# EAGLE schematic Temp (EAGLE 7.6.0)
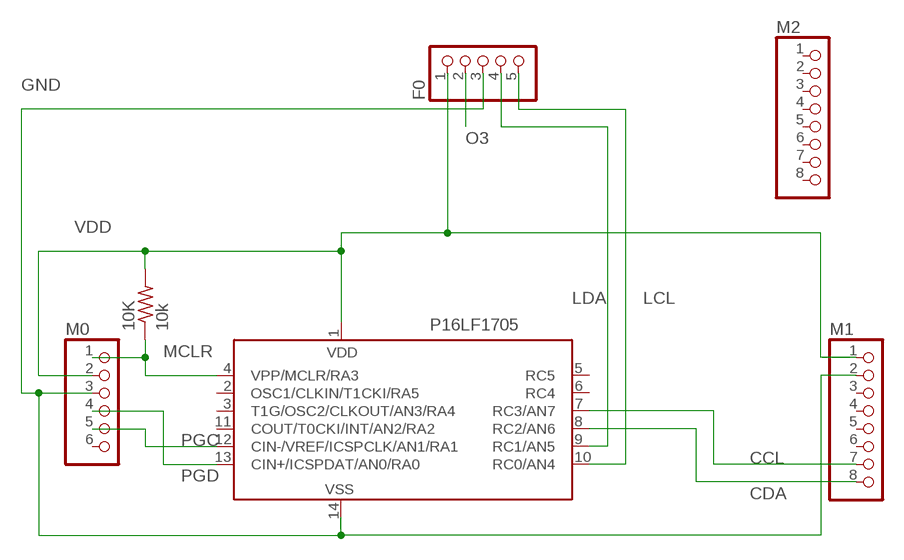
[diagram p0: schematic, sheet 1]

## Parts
10K  10k  R-US_0204/7  [0204/7]
F0  PINHD-1X5  [1X05]
M0  PINHD-1X6  [1X06]
M1  PINHD-1X8  [1X08]
M2  PINHD-1X8  [1X08]
P16LF1705  PIC16F676SL  [SO-14]

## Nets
CCL: M1.7 P16LF1705.7(RC3/AN7)
CDA: M1.8 P16LF1705.8(RC2/AN6)
GND: F0.3 M0.3 M1.2 P16LF1705.14(VSS)
LCL: F0.5 P16LF1705.10(RC0/AN4)
LDA: F0.4 P16LF1705.9(RC1/AN5)
MCLR: 10K.1 M0.1 P16LF1705.4(VPP/MCLR/RA3)
O3: F0.2
PGC: M0.5 P16LF1705.12(CIN-/VREF/ICSPCLK/AN1/RA1)
PGD: M0.4 P16LF1705.13(CIN+/ICSPDAT/AN0/RA0)
VDD: 10K.2 F0.1 M0.2 M1.1 P16LF1705.1(VDD)
Unconnected: M0.6 M1.3 M1.4 M1.5 M1.6 M2.1 M2.2 M2.3 M2.4 M2.5 M2.6 M2.7 M2.8 P16LF1705.2(OSC1/CLKIN/T1CKI/RA5) P16LF1705.3(T1G/OSC2/CLKOUT/AN3/RA4) P16LF1705.5(RC5) P16LF1705.6(RC4) P16LF1705.11(COUT/T0CKI/INT/AN2/RA2)

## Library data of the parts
10K = adafruit:R-US_: RESISTOR, American symbol
F0 = pinhead:PINHD-1X5: PIN HEADER
M0 = pinhead:PINHD-1X6: PIN HEADER
M1 M2 = pinhead:PINHD-1X8: PIN HEADER
P16LF1705 = microchip:PIC16F676: 14-Pin, Flash-Based 8-Bit CMOS Microcontroller High Performance RISC CPU: * Only 35 instructions to learn - All single-cycle instructions except branches * Operating speed: - DC - 20 MHz oscillator/clock input - DC - 200 ns instruction cycle * Internal and external oscillator options - Precision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; MF: MICROCHIP; MPN: PIC16F676-I/SL; OC_FARNELL: 9760520; OC_NEWARK: 92C4557

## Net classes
0 default: width 0.305 mm, drill 0.61 mm, clearance 0.254 mm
